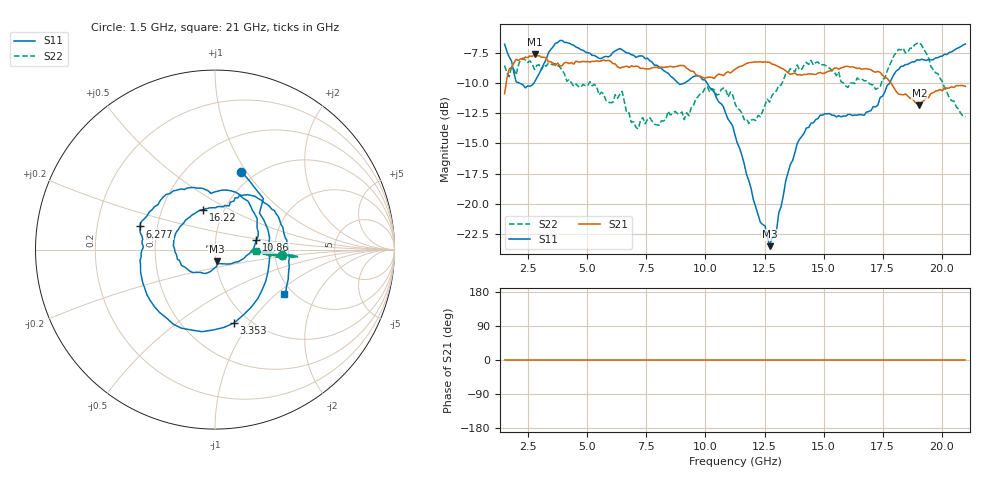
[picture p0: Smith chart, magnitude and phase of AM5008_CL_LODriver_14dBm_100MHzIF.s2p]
!Keysight Technologies,N5245B,MY58422270,A.16.20.02
!Mixer S2P File: Scalar Mixer Measurement
!Calibration State: On
!Parameters: Stimulus Freq, S11, SC21, SC12, S22
# Hz  S  DB  R  50.0
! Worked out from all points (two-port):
!   201 points, 1.5 GHz to 21 GHz, reference 50 ohm
!   highest |S21| = -7.60 dB at 2.768 GHz (marker M1); lowest = -11.8 dB at 19.05 GHz (marker M2)
!   |S21| within 3 dB of the highest: 1.521 GHz to 18.05 GHz (16.52 GHz wide, 169 % of centre); 20.03 GHz to end of sweep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
!   lowest |S11| = -23.5 dB at 12.71 GHz (marker M3), VSWR 1.14, Z = 50.6 - j6.69 ohm
!   |S11| at or under -10 dB: 2.146 GHz to 2.728 GHz (582.2 MHz wide, 23.9 % of centre); 8.856 GHz to 9.094 GHz (238.7 MHz wide, 2.66 % of centre); 10.07 GHz to 17.79 GHz (7.714 GHz wide, 55.4 % of centre)
!   |S22| runs from -13.8 to -6.6 dB; largest |S21 - S12| = 0.42
!   S11 on the Smith chart (normalised r, x): 1.5 GHz: 0.86, +0.95; 3.353 GHz: 0.85, -0.85; 6.277 GHz: 0.40, +0.13; 10.86 GHz: 1.59, +0.18; 16.22 GHz: 0.80, +0.38; 21 GHz: 1.80, -1.14
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1.5e9  -6.76 71.3  -10.87 0.0  -200.00 90.0  -8.53 -4.5
1.9875e9  -9.88 39.4  -8.00 0.0  -200.00 90.0  -9.31 -6.9
2.7675e9  -9.90 -22.7  -7.60 0.0  -200.00 90.0  -8.86 -6.0
3.3525e9  -7.48 -75.5  -8.20 0.0  -200.00 90.0  -8.32 -4.5
3.645e9  -6.69 -99.0  -8.53 0.0  -200.00 90.0  -8.35 -6.1
4.1325e9  -6.61 -131.5  -8.27 0.0  -200.00 90.0  -9.84 -4.2
4.815e9  -7.26 -163.0  -8.18 0.0  -200.00 90.0  -10.10 -6.5
6.2775e9  -7.21 162.8  -8.62 0.0  -200.00 90.0  -11.26 -4.4
7.0575e9  -7.86 141.7  -8.58 0.0  -200.00 90.0  -13.67 -0.6
8.0325e9  -8.64 110.9  -8.75 0.0  -200.00 90.0  -13.49 -4.8
9.69e9  -9.37 70.5  -9.37 0.0  -200.00 90.0  -11.10 -4.1
1.086e10  -12.53 13.0  -9.15 0.0  -200.00 90.0  -10.50 -5.1
1.125e10  -14.30 -6.6  -8.85 0.0  -200.00 90.0  -11.67 -4.4
1.1835e10  -18.08 -37.3  -8.30 0.0  -200.00 90.0  -13.34 -3.8
1.27125e10  -23.53 -80.9  -8.26 0.0  -200.00 90.0  -11.57 -5.5
1.38825e10  -15.01 -133.8  -9.30 0.0  -200.00 90.0  -8.49 -3.6
1.4565e10  -13.28 -172.4  -9.25 0.0  -200.00 90.0  -8.47 -6.0
1.62225e10  -12.68 106.0  -8.62 0.0  -200.00 90.0  -9.98 -5.9
1.71975e10  -11.96 75.5  -9.08 0.0  -200.00 90.0  -10.51 -5.0
1.77825e10  -10.02 66.1  -9.83 0.0  -200.00 90.0  -8.53 -5.4
1.905e10  -8.08 30.8  -11.82 0.0  -200.00 90.0  -6.63 -5.8
2.1e10  -6.74 -32.7  -10.25 0.0  -200.00 90.0  -12.79 -1.7
